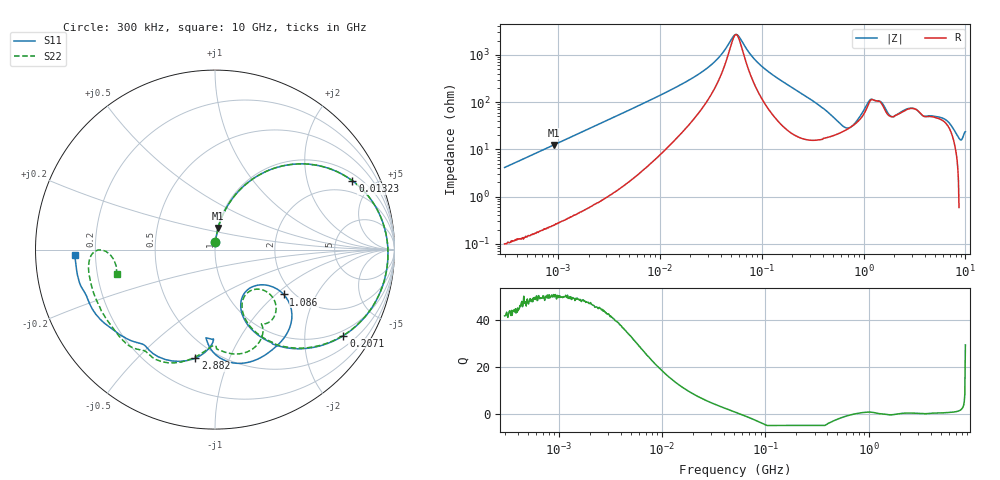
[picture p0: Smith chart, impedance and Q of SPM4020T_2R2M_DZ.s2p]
! S-Parameter Data Generated by TDK Corporation
! Copyright(C) 2024 TDK Corporation.
! All Rights Reserved.
! TDK P/N: SPM4020T-2R2M-DZ (SMD / SMT Inductor (Coil))
! Property: L=2.2uH at 100kHz
! Size(LxWxT): 4.3x4.1x2mm
! Model Type: s2p (Touchstone File Format Version 1.0)
! Frequency: DC=Yes Start=0.3MHz Stop=10000MHz 802points Log-sweep
! Model Generated on May 28, 2024
! Terms and conditions regarding TDK Simulation Models:
! 1)This simulation model is being provided solely for informational
!  purposes. Please refer to the specifications of the products in
!  terms of detailed characteristics of such products.
! 2)In no event shall TDK Corporation of any of its subsidiaries be
!  liable for any loss or damage arising, directly or indirectly,
!  from any information contained in this simulation model, including,
!  but not limited to loss or damages arising from any inaccuracies,
!  omissions or errors in connection with such information.
! 3)Any and all copyrights on this simulation model are owned by
!  TDK Corporation.  Duplication or redistribution of this simulation
!  model without prior written permission from TDK Corporation
!  is prohibited.
! 4)This simulation model is subject to any modification or change
!  without any prior notice.
! 5)Neither TDK Corporation nor any of its subsidiaries shall make any
!  warranty, express or implied, including but not limited to the
!  correctness, implied warranties of merchantability and fitness for
!  a particular purpose with respect to this simulation models.
! 6)The use of this simulation model shall be deemed to have consented
!  to the terms and conditions hereof.
! Port Assignments:
!  1 ---@@@--- 2
! Applicable Conditions:
!  Temperature = 25 degC
!  DC Bias Current = 0 A
!  Small Signal Operation
# Hz S MA R 50
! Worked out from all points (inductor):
!   801 points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, 300 kHz to 10 GHz, reference 50 ohm
!   read as one part in series: L = 2.18 uH near 318.3 kHz
!   highest Q = 50.1 at 905.9 kHz (marker M1), where L = 2.16 uH
!   self-resonance near 56.06 MHz
!   S11 on the Smith chart (normalised r, x): 300 kHz: 1.00, +0.08; 13.23 MHz: 1.32, +3.79; 207.1 MHz: 0.83, -3.09; 1.086 GHz: 1.78, -1.13; 2.882 GHz: 0.39, -0.76; 10 GHz: 0.12, -0.02
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300000  0.04156 86.5  0.9981 -2.3  0.9977 -2.3  0.04171 86.8
905948  0.1218 81.8  0.9901 -7.0  0.99 -7.0  0.1219 81.9
1713600  0.2245 75.8  0.9698 -13.0  0.9698 -13.0  0.2246 75.8
3822232  0.4531 61.4  0.8796 -27.1  0.8798 -27.1  0.4531 61.4
9671944  0.7803 35.4  0.5856 -51.6  0.5857 -51.6  0.7802 35.4
1.322782e7  0.8561 26.6  0.458 -59.2  0.4581 -59.2  0.856 26.7
3.162388e7  0.9514 7.5  0.1582 -69.1  0.1582 -69.1  0.9515 7.6
5.477226e7  0.9642 -1.9  0.03616 -11.5  0.03617 -11.5  0.9643 -1.9
1.050124e8  0.9505 -14.5  0.1789 64.7  0.1789 64.7  0.9506 -14.4
2.070906e8  0.8613 -33.8  0.4275 50.5  0.4275 50.5  0.8614 -33.6
3.126428e8  0.7274 -49.5  0.5976 33.4  0.5976 33.4  0.7271 -49.0
6.407886e8  0.3657 -66.6  0.7534 -7.3  0.7534 -7.3  0.3662 -65.5
8.643532e8  0.2897 -47.4  0.7005 -28.9  0.7006 -28.9  0.3069 -46.9
1.085776e9  0.4569 -33.1  0.5129 -46.5  0.513 -46.5  0.4617 -42.6
1.418928e9  0.6539 -67.5  0.4057 -34.2  0.4058 -34.2  0.5291 -59.6
1.767019e9  0.556 -92.3  0.5097 -35.6  0.5097 -35.6  0.5841 -81.9
2.172958e9  0.4995 -91.0  0.5031 -55.5  0.5031 -55.5  0.5357 -91.1
2.882439e9  0.6148 -100.3  0.3761 -72.3  0.3762 -72.3  0.6158 -101.3
5.849356e9  0.7174 -140.5  0.2578 -111.3  0.2578 -111.3  0.7204 -137.2
8.09931e9  0.7623 -160.9  0.1815 -147.4  0.1815 -147.5  0.7166 -165.3
9.217363e9  0.7794 -169.6  0.1323 -161.9  0.1325 -161.8  0.6683 -179.2
1e10  0.7822 -178.0  0.1062 -157.9  0.1063 -158.1  0.5629 -166.1
